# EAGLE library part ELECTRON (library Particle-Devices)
The Particle Electron is a tiny development kit for creating cellular-connected electronics projects and products. It comes with a SIM card (Nano 4FF) and an affordable data plan for low-bandwidth things. Design files : here Product Page : Datasheet Github : Particle devices library
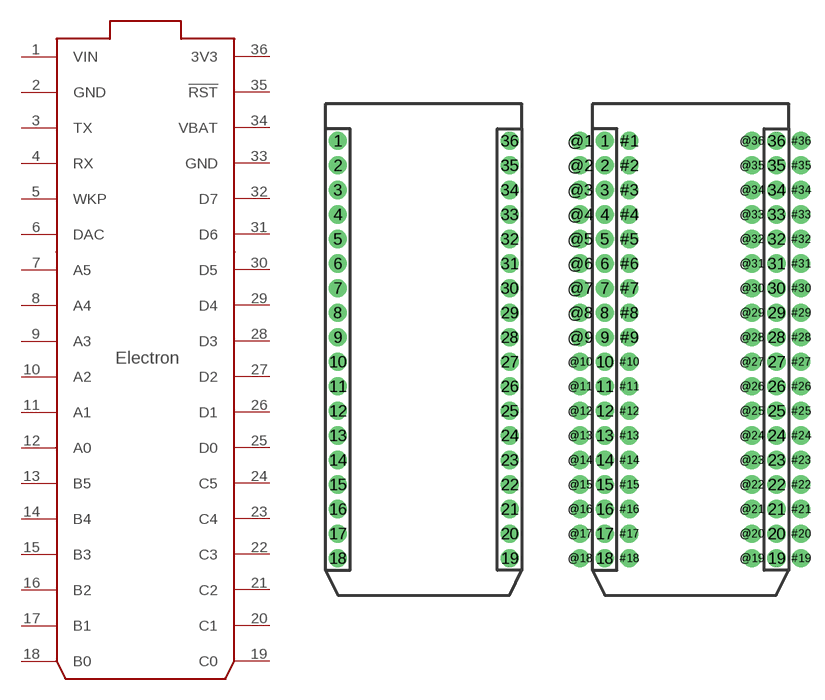
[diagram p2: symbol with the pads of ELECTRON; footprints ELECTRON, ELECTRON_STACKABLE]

Designator prefix -

## ELECTRON_WITH_HEADERS  [ELECTRON]
1  VIN  pwr
2  GND  pwr
3  TX
4  RX
5  WKP
6  DAC
7  A5
8  A4
9  A3
10  A2
11  A1
12  A0
13  B5
14  B4
15  B3
16  B2
17  B1
18  B0
19  C0
20  C1
21  C2
22  C3
23  C4
24  C5
25  D0
26  D1
27  D2
28  D3
29  D4
30  D5
31  D6
32  D7
33  GND  pwr
34  VBAT  pwr
35  !RST
36  3V3  pwr

## ELECTRON_WITH_STACKABLE_HEADERS  [ELECTRON_STACKABLE]
1  VIN  pwr
2  GND  pwr
3  TX
4  RX
5  WKP
6  DAC
7  A5
8  A4
9  A3
10  A2
11  A1
12  A0
13  B5
14  B4
15  B3
16  B2
17  B1
18  B0
19  C0
20  C1
21  C2
22  C3
23  C4
24  C5
25  D0
26  D1
27  D2
28  D3
29  D4
30  D5
31  D6
32  D7
33  GND  pwr
34  VBAT  pwr
35  !RST
36  3V3  pwr
#1  VIN  pwr
#2  GND  pwr
#3  TX
#4  RX
#5  WKP
#6  DAC
#7  A5
#8  A4
#9  A3
#10  A2
#11  A1
#12  A0
#13  B5
#14  B4
#15  B3
#16  B2
#17  B1
#18  B0
#19  C0
#20  C1
#21  C2
#22  C3
#23  C4
#24  C5
#25  D0
#26  D1
#27  D2
#28  D3
#29  D4
#30  D5
#31  D6
#32  D7
#33  GND  pwr
#34  VBAT  pwr
#35  !RST
#36  3V3  pwr
@1  VIN  pwr
@2  GND  pwr
@3  TX
@4  RX
@5  WKP
@6  DAC
@7  A5
@8  A4
@9  A3
@10  A2
@11  A1
@12  A0
@13  B5
@14  B4
@15  B3
@16  B2
@17  B1
@18  B0
@19  C0
@20  C1
@21  C2
@22  C3
@23  C4
@24  C5
@25  D0
@26  D1
@27  D2
@28  D3
@29  D4
@30  D5
@31  D6
@32  D7
@33  GND  pwr
@34  VBAT  pwr
@35  !RST
@36  3V3  pwr

## Footprint ELECTRON (pad centres in mm)
drill 1.016 pad 1.88: 1 1.27,46.99; 2 1.27,44.45; 3 1.27,41.91; 4 1.27,39.37; 5 1.27,36.83; 6 1.27,34.29; 7 1.27,31.75; 8 1.27,29.21; 9 1.27,26.67; 10 1.27,24.13; 11 1.27,21.59; 12 1.27,19.05; 13 1.27,16.51; 14 1.27,13.97; 15 1.27,11.43; 16 1.27,8.89; 17 1.27,6.35; 18 1.27,3.81; 19 19.05,3.81; 20 19.05,6.35; 21 19.05,8.89; 22 19.05,11.43; 23 19.05,13.97; 24 19.05,16.51; 25 19.05,19.05; 26 19.05,21.59; 27 19.05,24.13; 28 19.05,26.67; 29 19.05,29.21; 30 19.05,31.75; 31 19.05,34.29; 32 19.05,36.83; 33 19.05,39.37; 34 19.05,41.91; 35 19.05,44.45; 36 19.05,46.99

## Footprint ELECTRON_STACKABLE (pad centres in mm)
drill 1.016 pad 1.88: 1 1.27,46.99; 2 1.27,44.45; 3 1.27,41.91; 4 1.27,39.37; 5 1.27,36.83; 6 1.27,34.29; 7 1.27,31.75; 8 1.27,29.21; 9 1.27,26.67; 10 1.27,24.13; 11 1.27,21.59; 12 1.27,19.05; 13 1.27,16.51; 14 1.27,13.97; 15 1.27,11.43; 16 1.27,8.89; 17 1.27,6.35; 18 1.27,3.81; 19 19.05,3.81; 20 19.05,6.35; 21 19.05,8.89; 22 19.05,11.43; 23 19.05,13.97; 24 19.05,16.51; 25 19.05,19.05; 26 19.05,21.59; 27 19.05,24.13; 28 19.05,26.67; 29 19.05,29.21; 30 19.05,31.75; 31 19.05,34.29; 32 19.05,36.83; 33 19.05,39.37; 34 19.05,41.91; 35 19.05,44.45; 36 19.05,46.99; #1 3.81,46.99; #2 3.81,44.45; #3 3.81,41.91; #4 3.81,39.37; #5 3.81,36.83; #6 3.81,34.29; #7 3.81,31.75; #8 3.81,29.21; #9 3.81,26.67; #10 3.81,24.13; #11 3.81,21.59; #12 3.81,19.05; #13 3.81,16.51; #14 3.81,13.97; #15 3.81,11.43; #16 3.81,8.89; #17 3.81,6.35; #18 3.81,3.81; #19 21.59,3.81; #20 21.59,6.35; #21 21.59,8.89; #22 21.59,11.43; #23 21.59,13.97; #24 21.59,16.51; #25 21.59,19.05; #26 21.59,21.59; #27 21.59,24.13; #28 21.59,26.67; #29 21.59,29.21; #30 21.59,31.75; #31 21.59,34.29; #32 21.59,36.83; #33 21.59,39.37; #34 21.59,41.91; #35 21.59,44.45; #36 21.59,46.99; @1 -1.27,46.99; @2 -1.27,44.45; @3 -1.27,41.91; @4 -1.27,39.37; @5 -1.27,36.83; @6 -1.27,34.29; @7 -1.27,31.75; @8 -1.27,29.21; @9 -1.27,26.67; @10 -1.27,24.13; @11 -1.27,21.59; @12 -1.27,19.05; @13 -1.27,16.51; @14 -1.27,13.97; @15 -1.27,11.43; @16 -1.27,8.89; @17 -1.27,6.35; @18 -1.27,3.81; @19 16.51,3.81; @20 16.51,6.35; @21 16.51,8.89; @22 16.51,11.43; @23 16.51,13.97; @24 16.51,16.51; @25 16.51,19.05; @26 16.51,21.59; @27 16.51,24.13; @28 16.51,26.67; @29 16.51,29.21; @30 16.51,31.75; @31 16.51,34.29; @32 16.51,36.83; @33 16.51,39.37; @34 16.51,41.91; @35 16.51,44.45; @36 16.51,46.99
